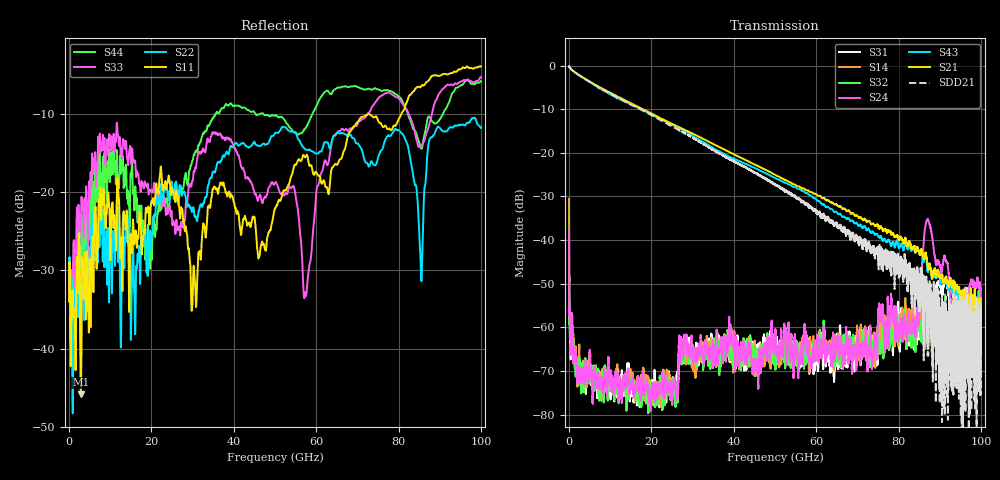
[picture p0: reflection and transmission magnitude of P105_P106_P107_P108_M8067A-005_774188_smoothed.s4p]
!Keysight Technologies PLTS 2021(64 bit), Build 20210202.1
!S11 smoothed in format LOGMAG, average points = 21
!S12 smoothed in format LOGMAG, average points = 21
!S13 smoothed in format LOGMAG, average points = 21
!S14 smoothed in format LOGMAG, average points = 21
!S21 smoothed in format LOGMAG, average points = 21
!S22 smoothed in format LOGMAG, average points = 21
!S23 smoothed in format LOGMAG, average points = 21
!S24 smoothed in format LOGMAG, average points = 21
!S31 smoothed in format LOGMAG, average points = 21
!S32 smoothed in format LOGMAG, average points = 21
!S33 smoothed in format LOGMAG, average points = 21
!S34 smoothed in format LOGMAG, average points = 21
!S41 smoothed in format LOGMAG, average points = 21
!S42 smoothed in format LOGMAG, average points = 21
!S43 smoothed in format LOGMAG, average points = 21
!S44 smoothed in format LOGMAG, average points = 21
!$DUT_CFG_DESC: Default 4-Port Configuration
!$NUMBER_PORTS: 4
!$DIFF_PORT_MAP: 1|2P|2|2P|0|UC|0|UC|
!$PORT_MAP: 1|1|<<<<<<|2|2|>>>>>>|3|3|<<<<<<|4|4|>>>>>>|
!Date: Monday, December 04, 2023, 05:48:59
!S4P File: Measurements: <S11,S12,S13,S14>,
!<S21,S22,S23,S24>,
!<S31,S32,S33,S34>,
!<S41,S42,S43,S44>:
# MHz S  RI  R 50
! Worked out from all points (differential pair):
!   10000 points, 10 MHz to 100 GHz, reference 50 ohm
!   strongest paths, dB at 10 MHz, 25.01 GHz, 50.01 GHz, 75.01 GHz, 100 GHz:
!     S21: -0.1, -13.4, -25.0, -36.6, -53.4
!     S43: -0.3, -13.6, -25.8, -39.1, -66.5
!     S24: -37.7, -77.0, -63.7, -58.2, -55.5
!     S32: -52.2, -73.2, -65.7, -61.4, -70.0
!     S14: -30.5, -76.3, -68.3, -61.8, -59.0
!     S31: -47.8, -73.1, -66.1, -63.9, -60.4
!   taken as a pair (ports 1,3 in; 2,4 out), SDD21 dB: -0.4, -14.0, -27.2, -41.9, -66.4
!   lowest |S11| = -45.8 dB at 2.85 GHz (marker M1), VSWR 1.01, Z = 50.1 + j0.5 ohm
!   |S11| at or under -10 dB: start of sweep to 80.73 GHz
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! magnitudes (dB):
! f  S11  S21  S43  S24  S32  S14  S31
! 10 MHz  -34.0  -0.1  -0.3  -37.7  -52.2  -30.5  -47.8
! 2.85 GHz  -45.8  -2.5  -2.5  -70.9  -72.9  -69.5  -71.1
! 57.36 GHz  -15.6  -28.5  -29.1  -62.1  -64.8  -68.1  -67.5
! 72.81 GHz  -10.1  -35.6  -37.5  -64.5  -62.4  -68.5  -60.5
! 83.95 GHz  -6.9  -41.9  -42.8  -58.9  -64.3  -58.3  -62.6
! 87.06 GHz  -5.9  -45.9  -47.3  -35.2  -60.9  -63.6  -59.3
! 100 GHz  -4.0  -53.4  -66.5  -55.5  -70.0  -59.0  -60.4
